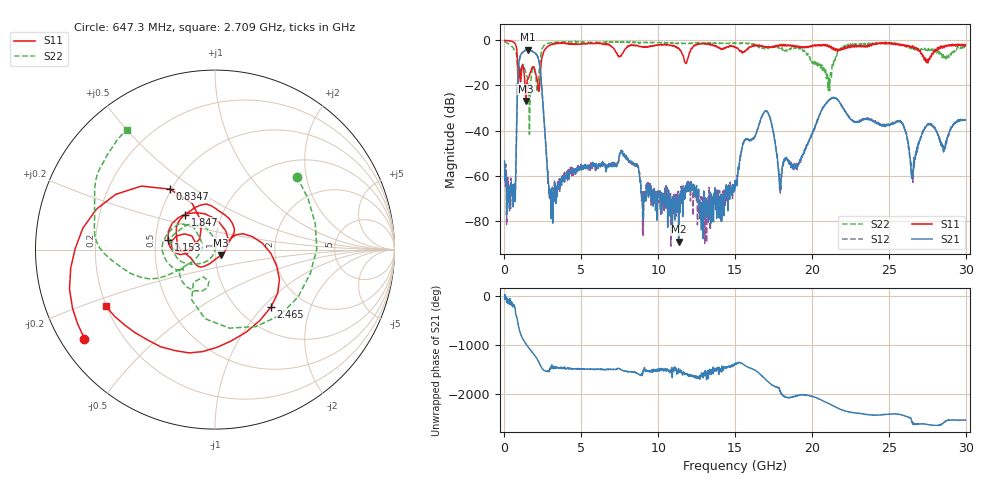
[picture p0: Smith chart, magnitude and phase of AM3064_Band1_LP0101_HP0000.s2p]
# Hz S DB R 50.0
!freq dBS11 angS11 dBS21 angS21 dBS12 angS12 dBS22 angS22
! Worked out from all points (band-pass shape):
!   1600 points, 10 MHz to 29.98 GHz, reference 50 ohm
!   highest |S21| = -4.13 dB at 1.528 GHz (marker M1); lowest = -89.4 dB at 11.33 GHz (marker M2)
!   |S21| within 3 dB of the highest: 1.02 GHz to 2.153 GHz (1.133 GHz wide, 71.4 % of centre)
!   lowest |S11| = -26.9 dB at 1.397 GHz (marker M3), VSWR 1.10, Z = 53.2 - j3.46 ohm
!   |S11| at or under -10 dB: 848.7 MHz to 2.392 GHz (1.544 GHz wide, 95.3 % of centre); 11.7861 GHz to 11.83828 GHz (52.18 MHz wide, 0.442 % of centre)
!   |S22| runs from -41.8 to -0.4 dB; largest |S21 - S12| = 0.0082
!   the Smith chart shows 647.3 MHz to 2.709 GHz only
!   S11 on the Smith chart (normalised r, x): 647.3 MHz: 0.07, -0.31; 834.7 MHz: 0.49, +0.40; 1.153 GHz: 0.58, +0.07; 1.847 GHz: 0.67, +0.28; 2.465 GHz: 1.39, -1.11; 2.709 GHz: 0.20, -0.24
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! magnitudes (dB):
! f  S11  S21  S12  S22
! 10 MHz  0.0  -53.5  -60.9  -0.4
! 647.3 MHz  -1.1  -69.7  -69.4  -4.3
! 834.7 MHz  -7.5  -24.7  -24.6  -10.2
! 1.153 GHz  -11.4  -5.6  -5.5  -11.2
! 1.397 GHz  -26.9  -4.2  -4.2  -15.3
! 1.528 GHz  -17.2  -4.1  -4.1  -18.9
! 1.847 GHz  -11.8  -5.0  -4.9  -12.4
! 2.465 GHz  -7.0  -24.5  -24.5  -3.4
! 2.709 GHz  -3.3  -48.7  -48.1  -1.7
! 3.065 GHz  -1.8  -65.8  -74.6  -1.0
! 5.015 GHz  -1.4  -56.1  -56.3  -0.6
! 7.639 GHz  -6.1  -49.5  -49.6  -0.7
! 10 GHz  -2.0  -69.8  -68.2  -1.0
! 11.33 GHz  -3.5  -89.4  -70.5  -1.2
! 15 GHz  -3.0  -65.4  -64.5  -1.4
! 16.94 GHz  -2.8  -31.7  -31.5  -3.5
! 17.93 GHz  -2.1  -62.2  -67.9  -3.0
! 19.99 GHz  -2.8  -41.8  -41.8  -9.4
! 21.38 GHz  -3.2  -25.4  -25.4  -11.6
! 25 GHz  -1.0  -37.6  -37.3  -1.2
! 26.55 GHz  -2.4  -60.0  -59.6  -4.4
! 29.98 GHz  -1.8  -35.3  -35.7  -2.9
